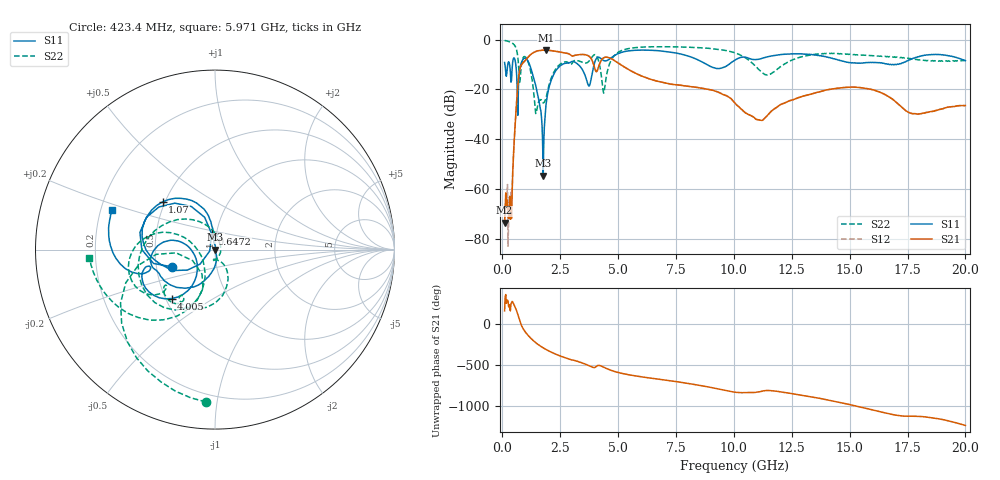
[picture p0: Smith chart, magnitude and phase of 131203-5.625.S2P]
!  2-Port S-parameters saved by WinCal
! VAR MeasName=S-Parameters (CALIBRATED_DATA) read from VNA (N5244A)
! VAR MeasDate=4/4/2013 3:57:13 PM
! VAR NAME=131203-5.625
! VAR FILENAME=131203-5.625.S2P
! VAR DATE=4/4/2013 3:57:13 PM
! VAR PHYS_PORTS=1,2
# Hz S MA R 50
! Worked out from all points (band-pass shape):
!   801 points, 100 MHz to 20 GHz, reference 50 ohm
!   highest |S21| = -4.26 dB at 1.891 GHz (marker M1); lowest = -73.4 dB at 100 MHz (marker M2)
!   |S21| within 3 dB of the highest: 1.098 GHz to 3.806 GHz (2.708 GHz wide, 110 % of centre); 4.398 GHz to 4.597 GHz (199.2 MHz wide, 4.43 % of centre)
!   lowest |S11| = -54.6 dB at 1.767 GHz (marker M3), VSWR 1.00, Z = 50.2 - j0.0584 ohm
!   |S11| at or under -10 dB: 1.177 GHz to 2.589 GHz (1.412 GHz wide, 75 % of centre); 3.278 GHz to 3.965 GHz (686.4 MHz wide, 19 % of centre); 8.834 GHz to 9.775 GHz (941.5 MHz wide, 10.1 % of centre)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
!   |S22| runs from -29.7 to -0.4 dB; largest |S21 - S12| = 0.0037
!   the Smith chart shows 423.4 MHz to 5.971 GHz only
!   S11 on the Smith chart (normalised r, x): 423.4 MHz: 0.61, -0.12; 647.2 MHz: 0.95, +0.17; 1.07 GHz: 0.49, +0.30; 4.005 GHz: 0.54, -0.34; 5.971 GHz: 0.25, +0.17
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1e8  0.3458 153.0  0.0002128 165.2  0.0003395 -150.3  0.9573 -22.2
3.4875e8  0.2227 142.3  0.00025 164.4  0.0003832 176.0  0.8877 -76.1
4.23375e8  0.2566 -158.0  0.0008044 -80.4  0.0009141 -37.3  0.8505 -93.4
6.4725e8  0.09035 102.0  0.08728 141.3  0.08738 141.2  0.5304 -159.6
8.4625e8  0.3635 -174.7  0.3221 -23.6  0.3228 -23.5  0.3592 -115.7
1.070125e9  0.3948 137.8  0.4184 -120.1  0.4195 -120.1  0.4001 177.0
1.44325e9  0.1204 96.2  0.5746 136.4  0.5762 136.4  0.0329 10.0
1.766625e9  0.001873 -18.1  0.6087 72.6  0.6101 72.5  0.05343 -95.4
1.891e9  0.05059 -78.8  0.6125 52.7  0.6143 52.6  0.06831 -68.2
2.413375e9  0.2718 -127.7  0.5698 -16.2  0.5719 -16.2  0.2956 -89.4
3.43325e9  0.2596 168.7  0.5014 -109.2  0.5025 -109.2  0.3515 -143.8
3.73175e9  0.1178 -164.2  0.4671 -142.8  0.4683 -142.9  0.3622 -140.9
4.005375e9  0.3648 -131.6  0.2541 -164.8  0.2552 -165.0  0.4974 -163.7
4.403375e9  0.3754 -165.6  0.435 -166.2  0.4371 -166.5  0.09231 -135.7
4.876e9  0.4864 -165.5  0.3707 142.4  0.3721 142.1  0.4967 -127.8
5.9705e9  0.6138 159.0  0.1892 80.9  0.1897 80.6  0.7015 -176.0
6.741625e9  0.5958 139.3  0.1448 51.0  0.1449 50.8  0.7178 163.2
1.005e10  0.3878 134.2  0.0532 -108.6  0.0536 -109.3  0.5409 90.6
1.1443e10  0.4506 118.2  0.02984 -87.1  0.02991 -87.4  0.1939 103.5
1.338325e10  0.4969 85.6  0.08192 -166.3  0.08142 -166.3  0.4954 111.5
1.669162e10  0.3189 75.7  0.07133 -10.3  0.07156 -10.4  0.4482 71.7
2e10  0.3779 36.8  0.04742 -153.7  0.04744 -153.6  0.3805 63.9
